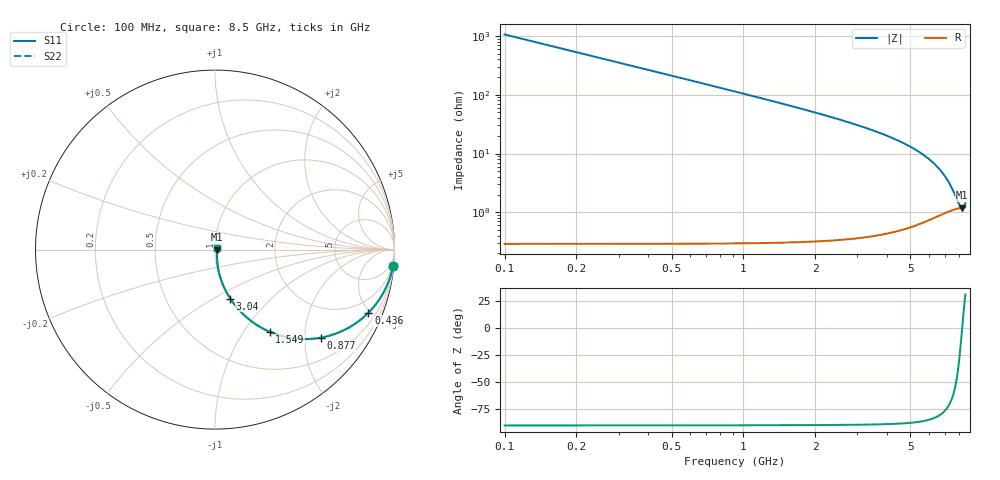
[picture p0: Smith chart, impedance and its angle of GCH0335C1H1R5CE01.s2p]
!Murata Part Number: GCH0335C1H1R5CE01
!These Parameters are Measured in Series Mode Connection
!Data Generated on Mar 13, 2026
!  o--ll--o
!Port1  Port2
!  o------o
!Operation Temp=25[degC], DC Bias Voltage=0[V]
!Freq. Start=100[MHz] Stop=9[GHz] 401[Steps]
# Hz S RI R 50
!Freq.(Hz) S11(Real) S11(Imag) S21(Real) S21(Imag) S12(Real) S12(Imag) S22(Real) S22(Imag)
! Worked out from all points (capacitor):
!   401 points, 100 MHz to 8.5 GHz, reference 50 ohm
!   read as one part in series: C = 1.5 pF near 142 MHz
!   lowest |Z| = 1.2 ohm at 8.227 GHz (marker M1)
!   series resonance near 8.238 GHz, so ESL is about 250 pH
!   S11 on the Smith chart (normalised r, x): 100 MHz: 1, -21; 436 MHz: 1.01, -4.85; 877 MHz: 1.01, -2.39; 1.549 GHz: 1.01, -1.32; 3.04 GHz: 1.01, -0.60; 8.5 GHz: 1.02, +0.01
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1e8  0.9912 -0.0934  0.00883 0.0934  0.00883 0.0934  0.9912 -0.0934
1.84e8  0.9707 -0.1684  0.0293 0.1684  0.0293 0.1684  0.9707 -0.1684
2.47e8  0.9484 -0.2209  0.0516 0.2209  0.0516 0.2209  0.9484 -0.2209
3.31e8  0.9108 -0.2845  0.0892 0.2845  0.0892 0.2845  0.9108 -0.2845
4.36e8  0.8545 -0.352  0.1455 0.352  0.1455 0.352  0.8545 -0.352
6.25e8  0.7397 -0.4379  0.2603 0.4379  0.2603 0.4379  0.7397 -0.4379
8.77e8  0.5882 -0.4909  0.4118 0.4909  0.4118 0.4909  0.5882 -0.4909
1.192e9  0.4315 -0.4936  0.5685 0.4936  0.5685 0.4936  0.4315 -0.4936
1.507e9  0.3167 -0.4629  0.6833 0.4629  0.6833 0.4629  0.3167 -0.4629
1.549e9  0.3041 -0.4577  0.6959 0.4577  0.6959 0.4577  0.3041 -0.4577
2.137e9  0.1775 -0.3786  0.8225 0.3786  0.8225 0.3786  0.1775 -0.3786
2.914e9  0.0938 -0.286  0.9062 0.286  0.9062 0.286  0.0938 -0.286
3.04e9  0.0851 -0.273  0.9149 0.273  0.9149 0.273  0.0851 -0.273
4.3e9  0.0345 -0.1698  0.9655 0.1698  0.9655 0.1698  0.0345 -0.1698
5.707e9  0.0152 -0.0911  0.9848 0.0911  0.9848 0.0911  0.0152 -0.0911
6.484e9  0.0118 -0.0577  0.9882 0.0577  0.9882 0.0577  0.0118 -0.0577
7.114e9  0.0111 -0.0345  0.9889 0.0345  0.9889 0.0345  0.0111 -0.0345
7.471e9  0.0112 -0.0227  0.9888 0.0227  0.9888 0.0227  0.0112 -0.0227
7.996e9  0.0117 -0.00681  0.9883 0.00681  0.9883 0.00681  0.0117 -0.00681
8.122e9  0.0118 -0.00323  0.9882 0.00323  0.9882 0.00323  0.0118 -0.00323
8.227e9  0.0119 -0.000302  0.9881 0.000302  0.9881 0.000302  0.0119 -0.000302
8.5e9  0.0121 0.00709  0.9879 -0.00709  0.9879 -0.00709  0.0121 0.00709
